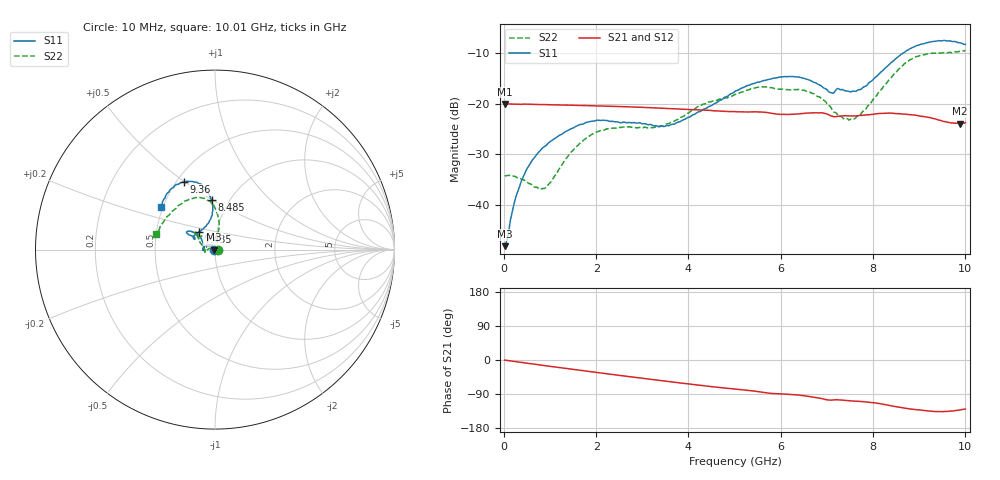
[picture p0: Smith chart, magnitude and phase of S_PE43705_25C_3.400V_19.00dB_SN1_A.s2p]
! Device ID: PE43705
! Serial: 1
! Insertion: A
! Impedance: 50 ohm
! Temp: 25C
! VDD: 3.400V
! Attenuation Step: 19.00dB
#  Hz  S  RI  R  50
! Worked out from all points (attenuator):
!   401 points, 10 MHz to 10.01 GHz, reference 50 ohm
!   highest |S21| = -20.04 dB at 10 MHz (marker M1); lowest = -23.9 dB at 9.885 GHz (marker M2)
!   lowest |S11| = -48.2 dB at 10 MHz (marker M3), VSWR 1.01, Z = 49.6 + j0.046 ohm
!   |S11| at or under -10 dB: start of sweep to 8.66 GHz
!   |S22| runs from -37.0 to -9.4 dB; largest |S21 - S12| = 0.001
!   S11 on the Smith chart (normalised r, x): 10 MHz: 0.99, +0.00; 7.435 GHz: 0.82, +0.16; 8.485 GHz: 0.83, +0.50; 9.36 GHz: 0.55, +0.50; 10.01 GHz: 0.49, +0.27
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1e7  -0.00388 0.000464  0.0995 -0.000402  0.0996 -0.000267  0.0193 0.000286
2.85e8  -0.00563 0.0119  0.0985 -0.00841  0.0985 -0.00834  0.017 0.00744
5.6e8  -0.0128 0.0219  0.0971 -0.0163  0.0972 -0.0162  0.0097 0.0129
9.1e8  -0.0277 0.0269  0.0945 -0.0259  0.0945 -0.0257  -0.00573 0.0138
1.685e9  -0.0602 0.0169  0.085 -0.0446  0.085 -0.0446  -0.0424 0.000212
2.26e9  -0.0676 0.000405  0.0756 -0.0566  0.0756 -0.0566  -0.0553 -0.0121
3.36e9  -0.0596 0.00352  0.0534 -0.0731  0.0534 -0.0729  -0.0588 0.00223
3.835e9  -0.0622 0.025  0.0431 -0.0771  0.043 -0.0771  -0.0699 0.0219
4.36e9  -0.073 0.051  0.0319 -0.0801  0.0319 -0.0802  -0.087 0.0484
5.01e9  -0.1 0.0866  0.0193 -0.0812  0.0194 -0.0812  -0.0987 0.0741
5.535e9  -0.1296 0.0997  0.00873 -0.0822  0.00877 -0.0822  -0.1119 0.0921
6.01e9  -0.153 0.1015  0.000838 -0.0784  0.00129 -0.0782  -0.1057 0.0905
6.685e9  -0.1442 0.0817  -0.0106 -0.0804  -0.0105 -0.0802  -0.0985 0.0794
7.085e9  -0.1109 0.0651  -0.0207 -0.0731  -0.0208 -0.0734  -0.0578 0.0727
7.435e9  -0.0919 0.0969  -0.0222 -0.0726  -0.0219 -0.0727  -0.0197 0.0688
7.76e9  -0.0483 0.1319  -0.0257 -0.072  -0.0254 -0.0721  0.00756 0.0812
8.36e9  -0.0122 0.2449  -0.0402 -0.07  -0.0399 -0.0701  0.0199 0.1727
8.485e9  -0.0181 0.2753  -0.0434 -0.0673  -0.0432 -0.0679  0.0124 0.2012
8.885e9  -0.0698 0.3551  -0.0502 -0.0591  -0.0493 -0.0593  -0.0463 0.2783
9.36e9  -0.1716 0.3765  -0.0508 -0.049  -0.0509 -0.0493  -0.1555 0.2742
9.885e9  -0.285 0.2816  -0.0422 -0.0475  -0.0426 -0.0474  -0.2996 0.1381
1.001e10  -0.3017 0.24  -0.0412 -0.0503  -0.0411 -0.0501  -0.3265 0.0844
